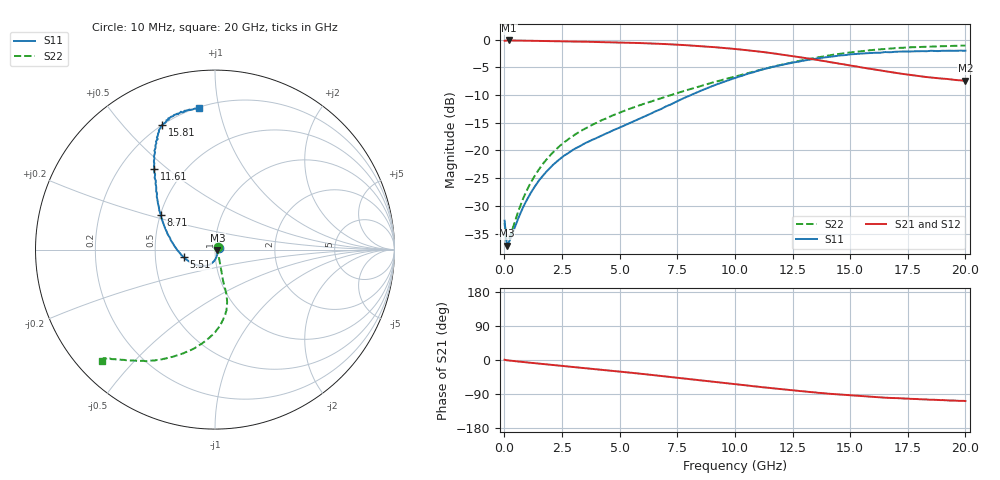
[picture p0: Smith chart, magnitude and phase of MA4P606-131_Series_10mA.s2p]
! AWR Design Environment (9226) Thu Aug 19 15:24:37 2021
! Document = '10mA'
! nPorts: 2, nXvals: 201
# GHz S DB R 50
!Freq DBS11 AngS11 DBS21 AngS21 DBS12 AngS12 DBS22 AngS22
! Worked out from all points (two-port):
!   201 points, 10 MHz to 20 GHz, reference 50 ohm
!   highest |S21| = -0.17 dB at 210 MHz (marker M1); lowest = -7.4 dB at 20 GHz (marker M2)
!   |S21| within 3 dB of the highest: start of sweep to 12.79 GHz
!   lowest |S11| = -37.2 dB at 110 MHz (marker M3), VSWR 1.03, Z = 51.4 - j0.331 ohm
!   |S11| at or under -10 dB: start of sweep to 8.104 GHz
!   |S22| runs from -37.3 to -1.1 dB; largest |S21 - S12| = 0.027
!   S11 on the Smith chart (normalised r, x): 10 MHz: 1.05, +0.01; 5.51 GHz: 0.70, -0.06; 8.71 GHz: 0.50, +0.22; 11.61 GHz: 0.34, +0.45; 15.81 GHz: 0.20, +0.64; 20 GHz: 0.21, +0.87
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0.01  -32.67 16.4  -0.23 0.7  -0.21 0.8  -33.09 37.5
0.11  -37.19 -13.5  -0.17 -0.8  -0.16 -0.7  -37.28 -14.6
0.21  -36.44 -25.2  -0.17 -1.4  -0.16 -1.4  -36.00 -26.2
0.51  -33.28 -51.0  -0.18 -3.4  -0.17 -3.3  -32.10 -48.9
0.81  -30.28 -66.9  -0.20 -5.3  -0.19 -5.1  -28.72 -58.4
1.11  -27.93 -77.5  -0.22 -7.2  -0.20 -7.0  -26.06 -63.9
1.41  -25.99 -85.5  -0.24 -9.0  -0.23 -8.7  -23.98 -67.1
1.91  -23.46 -96.7  -0.28 -12.0  -0.26 -11.7  -21.24 -70.3
2.41  -21.55 -106.6  -0.32 -14.9  -0.30 -14.6  -19.18 -72.7
3.41  -18.91 -125.9  -0.39 -20.9  -0.38 -20.4  -16.28 -74.8
4.41  -16.96 -145.2  -0.47 -26.9  -0.47 -26.3  -14.25 -75.5
5.51  -14.97 -166.0  -0.59 -33.7  -0.58 -32.9  -12.38 -75.4
6.71  -12.70 173.3  -0.77 -41.4  -0.75 -40.5  -10.71 -76.7
8.71  -8.93 147.6  -1.26 -54.8  -1.22 -53.5  -8.17 -83.2
10.01  -6.94 136.0  -1.70 -63.8  -1.65 -62.1  -6.70 -90.3
11.61  -4.98 126.8  -2.48 -74.4  -2.36 -72.8  -4.94 -102.3
13.41  -3.52 119.9  -3.57 -85.1  -3.43 -84.0  -3.35 -115.9
14.51  -2.89 116.2  -4.35 -91.0  -4.19 -90.0  -2.62 -123.2
15.81  -2.45 112.9  -5.25 -96.7  -5.15 -95.9  -1.96 -129.7
16.71  -2.29 110.0  -5.87 -100.0  -5.83 -99.2  -1.63 -132.6
19.01  -2.03 102.4  -7.05 -105.7  -7.20 -105.4  -1.22 -135.7
20  -2.01 96.4  -7.41 -108.3  -7.64 -107.1  -1.10 -135.4
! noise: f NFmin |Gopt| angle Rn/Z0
0.01  0  1  0  2e-20
2.21  0  1  0  2e-20
4.41  0  1  0  2e-20
6.61  0  1  0  2e-20
8.81  0  1  0  2e-20
11.11  0  1  0  2e-20
13.31  0  1  0  2e-20
15.51  0  1  0  2e-20
17.71  0  1  0  2e-20
20  0  1  0  2e-20
